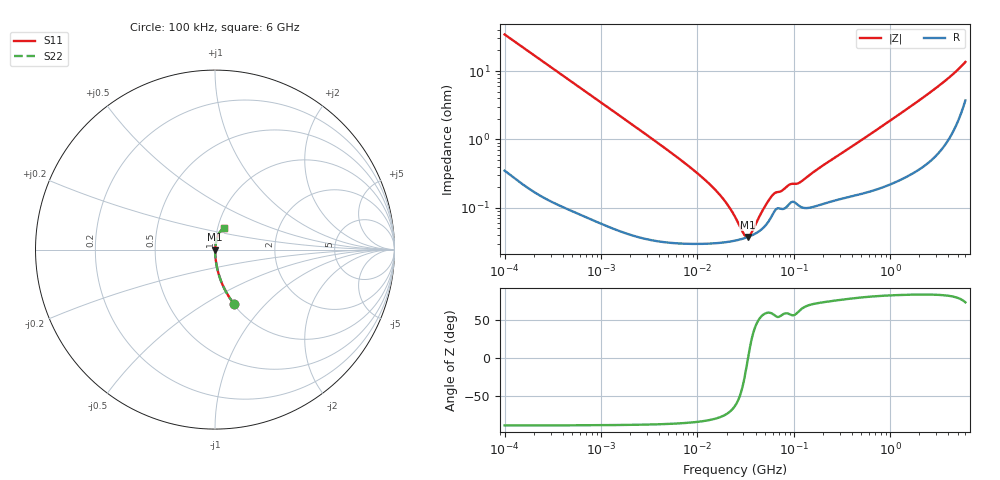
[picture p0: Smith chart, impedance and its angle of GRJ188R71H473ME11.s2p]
!Murata Part Number: GRJ188R71H473ME11
!These Parameters are Measured in Series Mode Connection
!Data Generated on Jun 19, 2026
!  o--ll--o
!Port1  Port2
!  o------o
!Operation Temp=25[degC], DC Bias Voltage=0[V]
!Freq. Start=100[kHz] Stop=6[GHz] 401[Steps]
# Hz S RI R 50
!Freq.(Hz) S11(Real) S11(Imag) S21(Real) S21(Imag) S12(Real) S12(Imag) S22(Real) S22(Imag)
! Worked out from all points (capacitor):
!   401 points, 100 kHz to 6 GHz, reference 50 ohm
!   read as one part in series: C = 46.4 nF near 105.7 kHz
!   lowest |Z| = 37.4 mohm at 33.15 MHz (marker M1)
!   series resonance near 33.41 MHz, so ESL is about 490 pH
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100000  0.1073 -0.3045  0.8927 0.3045  0.8927 0.3045  0.1073 -0.3045
151071  0.051 -0.215  0.949 0.215  0.949 0.215  0.051 -0.215
241130  0.0213 -0.1393  0.9787 0.1393  0.9787 0.1393  0.0213 -0.1393
631452  0.00375 -0.0545  0.9962 0.0545  0.9962 0.0545  0.00375 -0.0545
3987316  0.000397 -0.00863  0.9996 0.00863  0.9996 0.00863  0.000397 -0.00863
8379264  0.000313 -0.00391  0.9997 0.00391  0.9997 0.00391  0.000313 -0.00391
1.374747e7  0.000305 -0.00211  0.9997 0.00211  0.9997 0.00211  0.000305 -0.00211
1.912349e7  0.000315 -0.00123  0.9997 0.00123  0.9997 0.00123  0.000315 -0.00123
2.19429e7  0.000323 -0.000909  0.9997 0.000909  0.9997 0.000909  0.000323 -0.000909
2.517799e7  0.000335 -0.000603  0.9997 0.000603  0.9997 0.000603  0.000335 -0.000603
3.05238e7  0.000359 -0.000191  0.9996 0.000191  0.9996 0.000191  0.000359 -0.000191
3.314933e7  0.000374 -1.65e-05  0.9996 1.65e-05  0.9996 1.65e-05  0.000374 -1.65e-05
3.60007e7  0.000392 0.000159  0.9996 -0.000159  0.9996 -0.000159  0.000392 0.000159
4.872031e7  0.00052 0.000837  0.9995 -0.000837  0.9995 -0.000837  0.00052 0.000837
6.07118e7  0.00082 0.00133  0.9992 -0.00133  0.9992 -0.00133  0.00082 0.00133
7.565474e7  0.000963 0.00151  0.999 -0.00151  0.999 -0.00151  0.000963 0.00151
9.171783e7  0.00118 0.00187  0.9988 -0.00187  0.9988 -0.00187  0.00118 0.00187
1.142923e8  0.00106 0.00208  0.9989 -0.00208  0.9989 -0.00208  0.00106 0.00208
1.546735e8  0.00103 0.00306  0.999 -0.00306  0.999 -0.00306  0.00103 0.00306
9.76689e8  0.0025 0.0183  0.9975 -0.0183  0.9975 -0.0183  0.0025 0.0183
2.934752e9  0.00864 0.0546  0.9914 -0.0546  0.9914 -0.0546  0.00864 0.0546
6e9  0.0509 0.1195  0.9491 -0.1195  0.9491 -0.1195  0.0509 0.1195
